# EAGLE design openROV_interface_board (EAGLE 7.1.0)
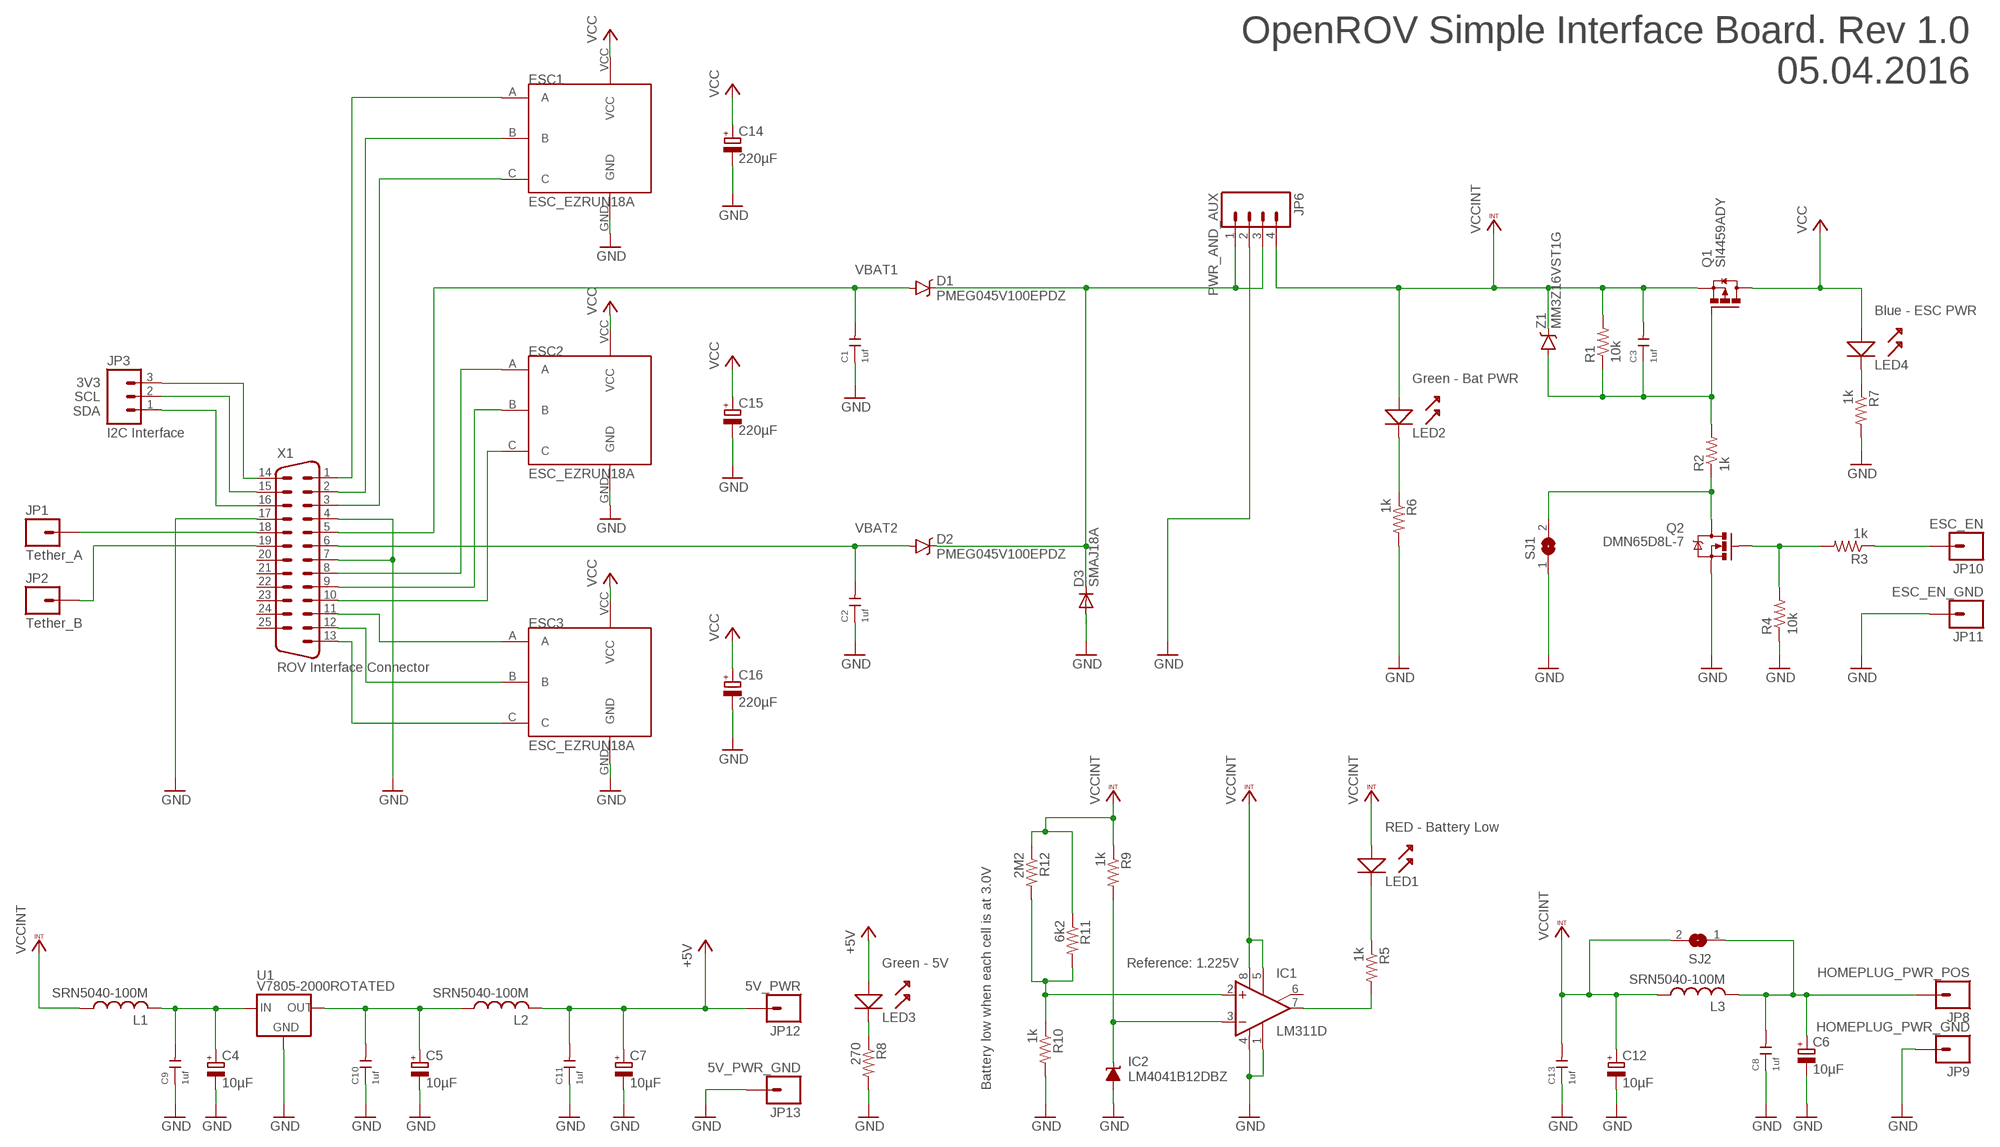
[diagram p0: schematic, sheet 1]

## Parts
C1  1uf  CERAMIC-1UF-25V-10%-X7R(0805)  [C0805]
C2  1uf  CERAMIC-1UF-25V-10%-X7R(0805)  [C0805]
C3  1uf  CERAMIC-1UF-25V-10%-X7R(0805)  [C0805]
C4  10µF  CPOL-EUE2-5  [E2-5]
C5  10µF  CPOL-EUE2-5  [E2-5]
C6  10µF  CPOL-EUE2-5  [E2-5]
C7  10µF  CPOL-EUE2-5  [E2-5]
C8  1uf  CERAMIC-1UF-25V-10%-X7R(0805)  [C0805]
C9  1uf  CERAMIC-1UF-25V-10%-X7R(0805)  [C0805]
C10  1uf  CERAMIC-1UF-25V-10%-X7R(0805)  [C0805]
C11  1uf  CERAMIC-1UF-25V-10%-X7R(0805)  [C0805]
C12  10µF  CPOL-EUE2-5  [E2-5]
C13  1uf  CERAMIC-1UF-25V-10%-X7R(0805)  [C0805]
C14  220µF  CPOL-EUE3.5-8  [E3,5-8]
C15  220µF  CPOL-EUE3.5-8  [E3,5-8]
C16  220µF  CPOL-EUE3.5-8  [E3,5-8]
D1  PMEG045V100EPDZ  [SOT1289]
D2  PMEG045V100EPDZ  [SOT1289]
D3  SMAJ18A  DIODE-DO-214AC  [DO-214AC]
ESC1  ESC_EZRUN18A  [ESC_EZRUN18A]
ESC2  ESC_EZRUN18A  [ESC_EZRUN18A]
ESC3  ESC_EZRUN18A  [ESC_EZRUN18A]
IC1  LM311D  [SO08]
IC2  LM4041B12DBZ  [DBZ_R-PDSO-G3]
JP1  Tether_A  M01PTH_LONGPAD  [1X01_LONGPAD]
JP2  Tether_B  M01PTH_LONGPAD  [1X01_LONGPAD]
JP3  I2C Interface  M03LONGPADS  [1X03_LONGPADS]
JP6  PWR_AND_AUX  M04LONGPADS  [1X04_LONGPADS]
JP8  HOMEPLUG_PWR_POS  M01PTH_LONGPAD  [1X01_LONGPAD]
JP9  HOMEPLUG_PWR_GND  M01PTH_LONGPAD  [1X01_LONGPAD]
JP10  ESC_EN  M01PTH_LONGPAD  [1X01_LONGPAD]
JP11  ESC_EN_GND  M01PTH_LONGPAD  [1X01_LONGPAD]
JP12  5V_PWR  M01PTH_LONGPAD  [1X01_LONGPAD]
JP13  5V_PWR_GND  M01PTH_LONGPAD  [1X01_LONGPAD]
L1  SRN5040-100M  [SRN5040_SERIES]
L2  SRN5040-100M  [SRN5040_SERIES]
L3  SRN5040-100M  [SRN5040_SERIES]
LED1  RED - Battery Low  LED-1206  [LED-1206]
LED2  Green - Bat PWR  LED-1206  [LED-1206]
LED3  Green - 5V  LED-1206  [LED-1206]
LED4  Blue - ESC PWR  LED-1206  [LED-1206]
Q1  SI4459ADY  [SO8]
Q2  DMN65D8L-7  [SOT-23]
R1  10k  R-US_M0805  [M0805]
R2  1k  R-US_M0805  [M0805]
R3  1k  R-US_M0805  [M0805]
R4  10k  R-US_M0805  [M0805]
R5  1k  R-US_M0805  [M0805]
R6  1k  R-US_M0805  [M0805]
R7  1k  R-US_M0805  [M0805]
R8  270  R-US_M0805  [M0805]
R9  1k  R-US_M0805  [M0805]
R10  1k  R-US_M0805  [M0805]
R11  6k2  R-US_M0805  [M0805]
R12  2M2  R-US_M0805  [M0805]
SJ1  SJW  [SJW]
SJ2  SJW  [SJW]
U1  V7805-2000ROTATED  [V78XX-2000R]
X1  ROV Interface Connector  DB25HP  [M25HP]
Z1  MM3Z16VST1G  [SOD-323]

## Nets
+5V: C7.+ C11.2 JP12.1 L2.P$2 LED3.1(A)
GND: C1.1 C2.1 C4.- C5.- C6.- C7.- C8.1 C9.1 C10.1 C11.1 C12.- C13.1 C14.- C15.- C16.- D3.A ESC1.GND ESC2.GND ESC3.GND IC1.1(GND) IC1.4(V-) IC2.2(A) JP6.2 JP9.1 JP11.1 JP13.1 Q2.2(S1) R4.1 R6.2 R7.2 R8.2 R10.2 SJ1.1 U1.P$2(GND) X1.4 X1.7 X1.17
N$1: JP1.1 X1.18
N$2: JP2.1 X1.19
N$3: JP3.3 X1.14
N$4: JP3.2 X1.15
N$5: JP3.1 X1.16
N$6: ESC3.C X1.13
N$7: ESC3.B X1.12
N$8: ESC3.A X1.11
N$9: ESC2.C X1.10
N$10: ESC2.B X1.9
N$11: ESC2.A X1.8
N$12: ESC1.A X1.1
N$13: ESC1.B X1.2
N$14: ESC1.C X1.3
N$15: D1.P$3(C) D2.P$3(C) D3.C JP6.1 JP6.3
N$16: C3.1 Q1.4(G) R1.1 R2.2 Z1.A
N$17: Q2.3(D1) R2.1 SJ1.2
N$18: Q2.1(G1) R3.2 R4.2
N$19: JP10.1 R3.1
N$20: C6.+ C8.2 JP8.1 L3.P$2 SJ2.1
N$21: C4.+ C9.2 L1.P$2 U1.P$1(IN)
N$22: C5.+ C10.2 L2.P$1 U1.P$3(OUT)
N$23: LED3.2(K) R8.1
N$24: IC1.3(-IN) IC2.1(C) R9.2
N$25: IC1.7(OUT) R5.2
N$26: LED1.2(K) R5.1
N$27: LED2.2(K) R6.1
N$28: LED4.2(K) R7.1
N$29: IC1.2(+IN) R10.1 R11.2 R12.2
VBAT1: C1.2 D1.P$1(A) D1.P$2(A) X1.5
VBAT2: C2.2 D2.P$1(A) D2.P$2(A) X1.6
VCC: C14.+ C15.+ C16.+ ESC1.VCC ESC2.VCC ESC3.VCC LED4.1(A) Q1.5(D) Q1.6(D) Q1.7(D) Q1.8(D)
VCCINT: C3.2 C12.+ C13.2 IC1.5(ON) IC1.8(V+) JP6.4 L1.P$1 L3.P$1 LED1.1(A) LED2.1(A) Q1.1(S) Q1.2(S) Q1.3(S) R1.2 R9.1 R11.1 R12.1 SJ2.2 Z1.C
Unconnected: IC1.6(ON/STR) X1.20 X1.21 X1.22 X1.23 X1.24 X1.25

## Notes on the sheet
- OpenROV Simple Interface Board. Rev 1.0
  05.04.2016
- 3V3
  SCL
  SDA
- Reference: 1.225V
- Battery low when each cell is at 3.0V

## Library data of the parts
C1-C3 C8-C11 C13 = Seeed-Capacitor-2016:CERAMIC-1UF-25V-10%-X7R(0805): 302010179; MOUSER: 603-CC805KKX7R8BB105; MPN: CC0805KKX7R8BB105
C4-C7 C12 = rcl:CPOL-EU: POLARIZED CAPACITOR, European symbol; MOUSER: 647-UPW1E100MDD
C14-C16 = rcl:CPOL-EU: POLARIZED CAPACITOR, European symbol; MOUSER: 661-EKZN350E221MH15D
D1 D2 = det_lib:PMEG045V100EPDZ; MOUSER: 771-PMEG045V100EPDZ
D3 = diode:DIODE-: DIODE; MOUSER: 511-SMAJ18A-TR
ESC1-ESC3 = uzzors2k:ESC_EZRUN18A
IC1 = linear:LM311: COMPARATOR; MOUSER: 511-LM311DT
IC2 = texas:LM4041: PRECISION MICROPOWER SHUNT VOLTAGE REFERENCE; MOUSER: 595-LM4041B12IDBZR; MPN: LM4041B12IDBZR; OC_FARNELL: 1575212; OC_NEWARK: 58K5882
JP1 JP2 JP8-JP13 = SparkFun-Connectors:M01: Header 1
JP3 = SparkFun-Connectors:M03: Header 3 Standard 3-pin 0.1" header. Use with straight break away headers (SKU : PRT-00116), right angle break away headers (PRT-00553), swiss pins (PRT-00743), machine pins (PRT-00117), and female headers (PRT-00115). Molex polarized connector foot print use with SKU : PRT-08232 with associated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
JP6 = SparkFun-Connectors:M04: Header 4 Standard 4-pin 0.1" header. Use with straight break away headers (SKU : PRT-00116), right angle break away headers (PRT-00553), swiss pins (PRT-00743), machine pins (PRT-00117), and female headers (PRT-00115). Molex polarized connector foot print use with SKU : PRT-08231 with associated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
L1-L3 = det_lib:SRN5040-100M; MOUSER: 652-SRN5040-100M
LED1 = uzzors2k:LED; MOUSER: 859-LTST-C230KRKT
LED2 LED3 = uzzors2k:LED; MOUSER: 859-LTST-C230KGKT
LED4 = uzzors2k:LED; MOUSER: 859-LTST-C230TBKT
Q1 = det_lib:SI4459ADY; MOUSER: 781-SI4459ADY-T1-GE3
Q2 = det_lib:DMN65D8L-7; MOUSER: 621-DMN65D8L-7
R1 R4 = rcl:R-US_: RESISTOR, American symbol; MOUSER: 71-CRCW0805-10K-E3
R2 R3 R5-R7 R9 R10 = rcl:R-US_: RESISTOR, American symbol; MOUSER: 588-AS08J1001ET
R8 = rcl:R-US_: RESISTOR, American symbol; MOUSER: 667-ERJ-6GEYJ271V
R11 = rcl:R-US_: RESISTOR, American symbol; MOUSER: 667-ERJ-6ENF6201V
R12 = rcl:R-US_: RESISTOR, American symbol; MOUSER: 603-RC0805FR-072M2L
SJ1 SJ2 = jumper:SJ: SMD solder JUMPER
U1 = det_lib:V7805-2000; MOUSER: 490-V7805-2000R
X1 = SparkFun-Connectors:DB25: Various DB25 connectors; MOUSER: 636-182-025-113R531
Z1 = det_lib:MM3Z16VST1G; MOUSER: 863-MM3Z16VST1G

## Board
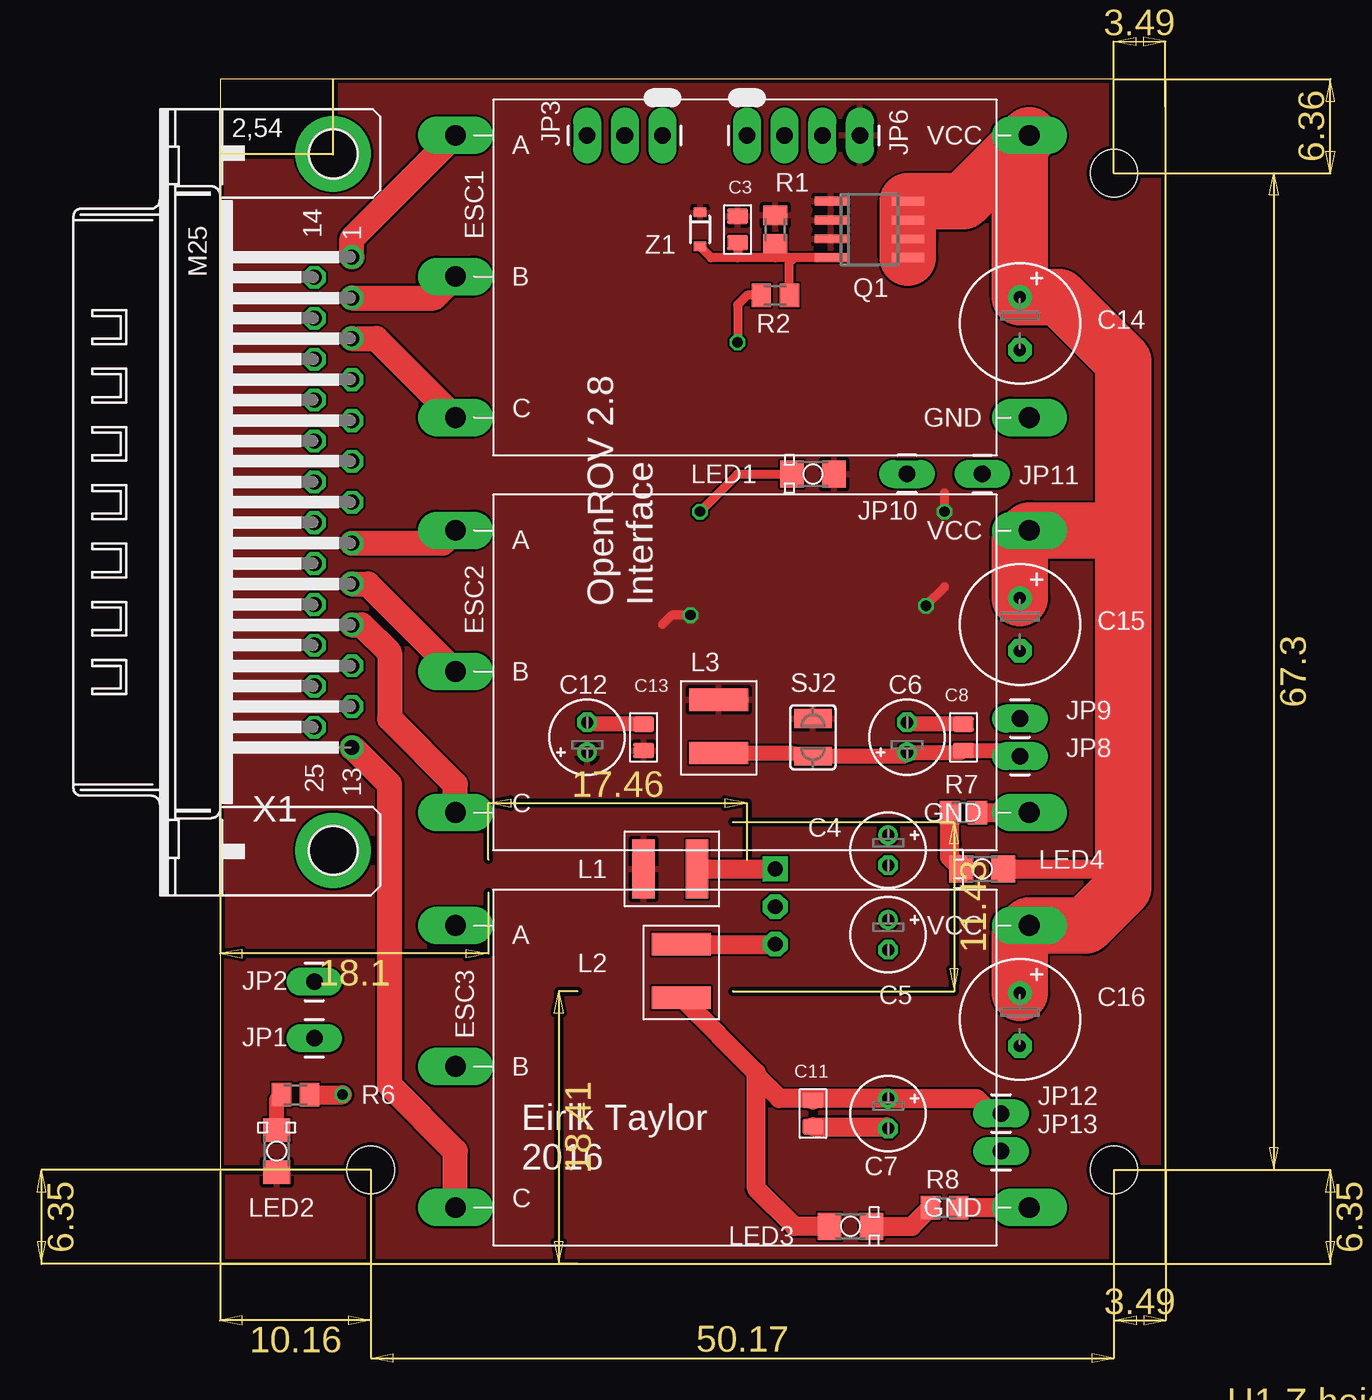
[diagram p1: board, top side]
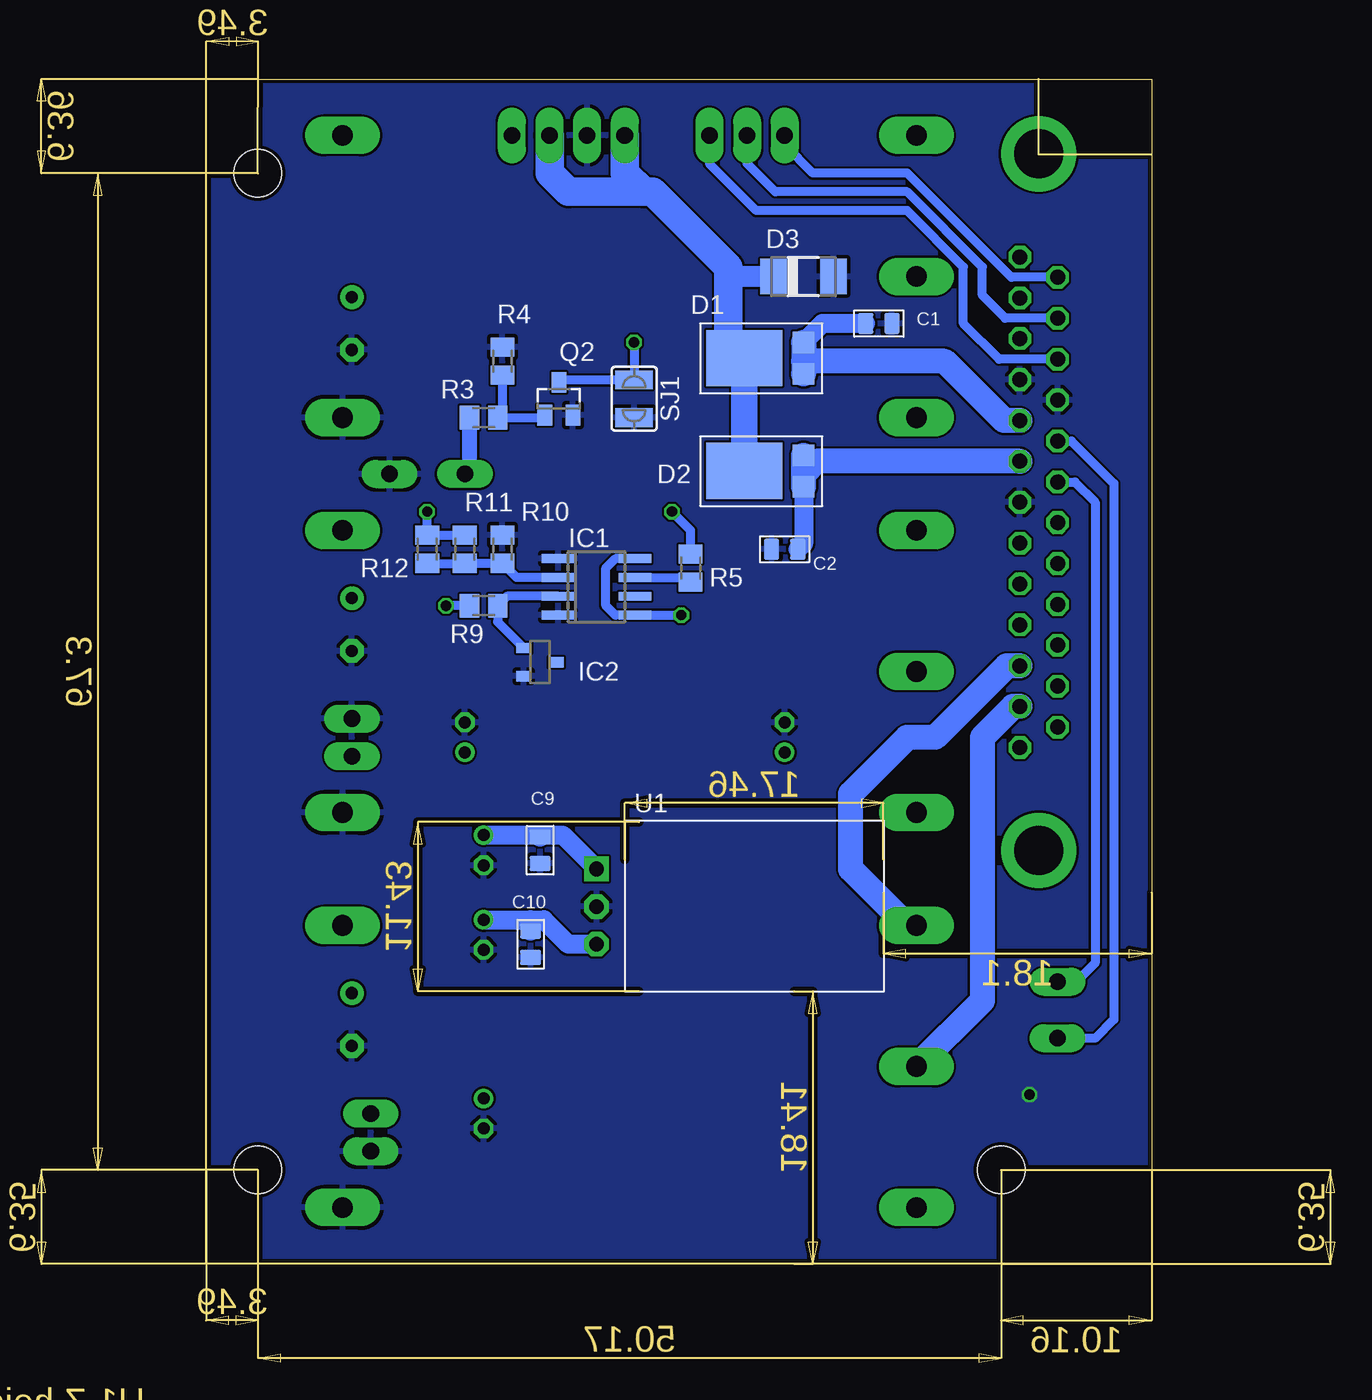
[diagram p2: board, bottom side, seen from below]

Size 87.59 x 89.49 mm. Coordinates in mm from the lower left corner, seen from the top.
Outline: 12.37,6.65 76.17,6.65 76.17,86.65 12.37,86.65 12.37,6.65
Copper layers (1*16): Top 0.035mm / dielectric 1.5mm / Bottom 0.035mm
Design rules "SeeedStudio_2layer_DRU_no_angle_20140221": minimum track width 6mil, minimum drill 12mil, track to track 6mil, track to pad 6mil, pad to pad 6mil, via to via 6mil, smd to smd 0mil, copper to edge 10mil, drill to drill 10mil, minimum pad ring 10mil, minimum via ring 6mil, stop-mask expansion 2mil, vias tented up to drill 100mil, thermal gap 10mil
Holes 3.2 mm at 22.53,13 72.69,13 72.69,80.3

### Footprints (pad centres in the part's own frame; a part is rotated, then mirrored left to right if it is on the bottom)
C0805 = smd 1.397 x 1.016: 1 0,0.889; 2 0,-0.889
E2-5 = drill 0.813 pad 1.27: + -1.016,0 | drill 0.813 pad 1.27 octagon: - 1.016,0
E3,5-8 = drill 0.813 pad 1.6: + -1.778,0 | drill 0.813 pad 1.6 octagon: - 1.778,0
SOT1289 = smd 1.44 x 1.44: P$1 -1.27,2.54; P$2 0.86,2.54 | smd 3.8 x 5.16: P$3 -0.205,-1.46
DO-214AC = smd 1.8 x 2.4: A 2.025,0; C -2.025,0
ESC_EZRUN18A = drill 1.4 pad 2.54 long: A -19.05,8.89; B -19.05,-0.635; C -19.05,-10.16; GND 19.685,-10.16; VCC 19.685,8.89
SO08 = smd 0.6 x 2.2: 1 -1.905,-2.6; 2 -0.635,-2.6; 3 0.635,-2.6; 4 1.905,-2.6; 5 1.905,2.6; 6 0.635,2.6; 7 -0.635,2.6; 8 -1.905,2.6
DBZ_R-PDSO-G3 = smd 0.7 x 1: 1 -0.95,-1.1; 2 0.95,-1.1; 3 0,1.1
1X01_LONGPAD = drill 1.118 pad 1.88 long: 1 0,0
1X03_LONGPADS = drill 1.118 pad 1.88 long: 1 0,0; 2 2.54,0; 3 5.08,0
1X04_LONGPADS = drill 1.118 pad 1.88 long: 1 0,0; 2 2.54,0; 3 5.08,0; 4 7.62,0
SRN5040_SERIES = smd 1.5 x 4: P$1 0,0; P$2 3.6,0
LED-1206 = smd 1.6 x 1.803: 1 -1.422,0; 2 1.422,0
SO8 = smd 0.6 x 2.2: 1 -1.905,-2.6; 2 -0.635,-2.6; 3 0.635,-2.6; 4 1.905,-2.6; 5 1.905,2.6; 6 0.635,2.6; 7 -0.635,2.6; 8 -1.905,2.6
SOT-23 = smd 1 x 1.4: 1 -0.95,-1.1; 2 0.95,-1.1; 3 0,1.1
M0805 = smd 1.3 x 1.6: 1 -0.95,0; 2 0.95,0
SJW = smd 1.27 x 2.54: 1 -1.27,0; 2 1.27,0
V78XX-2000R = drill 1 pad 1.676 square: P$1 -8.89,2.54 | drill 1 pad 1.676 octagon: P$2 -8.89,0; P$3 -8.89,-2.54
M25HP = drill 1.016 octagon: 1 -16.561,1.27; 2 -13.792,1.27; 3 -11.049,1.27; 4 -8.28,1.27; 5 -5.512,1.27; 6 -2.769,1.27; 7 0,1.27; 8 2.769,1.27; 9 5.512,1.27; 10 8.28,1.27; 11 11.049,1.27; 12 13.792,1.27; 13 16.561,1.27; 14 -15.189,-1.27; 15 -12.421,-1.27; 16 -9.652,-1.27; 17 -6.909,-1.27; 18 -4.14,-1.27; 19 -1.372,-1.27; 20 1.372,-1.27; 21 4.14,-1.27; 22 6.909,-1.27; 23 9.652,-1.27; 24 12.421,-1.27; 25 15.189,-1.27 | drill 3.302 pad 5.08: G1 -23.52,0; G2 23.52,0
SOD-323 = smd 0.63 x 0.83: A 1.15,0; C -1.15,0

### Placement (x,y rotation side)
C1  30.78,70.15 270 bottom
C2  37.13,54.91 90 bottom
C3  47.29,76.5 180 top
C4  57.45,34.59 270 top
C5  57.45,28.88 270 top
C6  58.72,42.21 90 top
C7  57.45,16.81 270 top
C8  62.53,42.21 0 top
C9  53.64,34.59 180 bottom
C10  54.27,28.24 180 bottom
C11  52.37,16.81 180 top
C12  37.13,42.21 90 top
C13  40.94,42.21 0 top
C14  66.34,70.15 270 top
C15  66.34,49.83 270 top
C16  66.34,23.16 270 top
D1  38.4,67.61 270 bottom
D2  38.4,59.99 270 bottom
D3  35.86,73.33 0 bottom
ESC1  47.29,73.96 0 top
ESC2  47.29,47.29 0 top
ESC3  47.29,20.62 0 top
IC1  49.83,52.37 270 bottom
IC2  53.64,47.29 270 bottom
JP1  18.72,21.89 90 top
JP2  18.72,25.7 90 top
JP3  42.21,82.85 180 top
JP6  47.93,82.85 0 top
JP8  66.34,40.94 90 top
JP9  66.34,43.48 90 top
JP10  58.72,59.99 270 top
JP11  63.8,59.99 90 top
JP12  65.07,16.81 90 top
JP13  65.07,14.27 90 top
L1  40.94,33.32 0 top
L2  43.48,28.24 270 top
L3  46.02,44.75 270 top
LED1  52.37,59.99 180 top
LED2  16.18,14.27 90 top
LED3  54.91,9.19 0 top
LED4  63.8,33.32 180 top
Q1  56.18,76.5 270 top
Q2  52.37,65.07 0 bottom
R1  49.83,76.5 90 top
R2  49.83,72.06 0 top
R3  57.45,63.8 0 bottom
R4  56.18,67.61 270 bottom
R5  43.48,53.64 270 bottom
R6  17.45,18.08 0 top
R7  62.53,37.13 0 top
R8  61.26,10.46 0 top
R9  57.45,51.1 0 bottom
R10  56.18,54.91 90 bottom
R11  58.72,54.91 270 bottom
R12  61.26,54.91 270 bottom
SJ1  47.29,65.07 90 bottom
SJ2  52.37,42.21 90 top
U1  40.94,30.78 0 bottom
X1  19.99,58.09 270 top
Z1  44.75,76.5 270 top

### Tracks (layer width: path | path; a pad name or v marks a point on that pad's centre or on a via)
+5V
  Top 1.27: 52.37,17.83 C7.+ 63.42,17.83 64.44,16.81 | L2.P$2 48.56,19.56 48.56,19.35 | C11.2 52.37,17.83 | JP12.1 64.44,16.81 | 64.44,16.81 63.8,16.81 | LED3.1 51.1,9.19 48.56,11.73 48.56,19.35 | 52.37,17.83 50.08,17.83 48.56,19.35
GND  (via drill 0.7)
  Top 1.016: C13.1 37.26,43.1 C12.- | C8.1 58.85,43.1 C6.-
  Top 1.27: C11.1 57.32,15.92 C7.- | R8.2 ESC3.GND | R6.2 v20.62,18.08 | R7.2 ESC2.GND
  pour Bottom: 12.37,86.66 100,86.66 100,6.65 12.37,6.65
N$1
  Bottom 0.61: X1.18 17.78,62.23 14.91,59.35 14.91,23.16 16.18,21.89 JP1.1
N$2
  Bottom 0.61: X1.19 17.55,59.46 16.18,58.09 16.18,26.97 17.45,25.7 JP2.1
N$3
  Bottom 0.61: X1.14 21.84,73.27 28.88,80.31 35.23,80.31 37.13,82.22 JP3.3
N$4
  Bottom 0.61: X1.15 22.25,70.51 23.8,72.06 23.8,73.96 28.88,79.04 37.77,79.04 39.67,80.95 JP3.2
N$5
  Bottom 0.61: X1.16 22.65,67.74 25.07,70.15 25.07,73.96 28.88,77.77 39.04,77.77 42.21,80.95 JP3.1
N$6
  Top 1.676: X1.13 21.31,41.52 23.8,39.03 23.8,18.71 28.24,14.27 ESC3.C
N$7
  Bottom 1.676: X1.12 21.71,44.29 23.8,42.21 23.8,24.43 ESC3.B
N$8
  Bottom 1.676: ESC3.A 28.88,29.51 32.69,33.32 32.69,38.4 28.88,42.21 26.97,42.21 22.14,47.04 X1.11
N$9
  Top 1.676: X1.10 21.92,49.8 23.8,47.92 23.8,43.48 28.24,39.03 ESC2.C
N$10
  Top 1.676: X1.9 22.32,52.57 ESC2.B
N$11
  Top 1.676: X1.8 27.38,55.32 ESC2.A
N$12
  Top 1.676: X1.1 21.26,75.87 ESC1.A
N$13
  Top 1.676: X1.2 26.79,71.88 ESC1.B
N$14
  Top 1.676: X1.3 22.91,69.13 ESC1.C
N$15
  Bottom 1.422: D3.C 40.31,73.33 40.94,73.96
  Bottom 1.778: D1.P$3 D2.P$3
  Bottom 1.93: D1.P$3 40.94,68.89 40.94,73.96 46.02,79.04 46.66,79.04 | 46.66,79.04 51.73,79.04 53.01,80.31 JP6.3 | JP6.1 47.93,80.31 46.66,79.04
N$16
  Top 0.61: Q1.4 51.1,74.59 | 51.1,74.59 49.83,74.59 | 49.83,74.59 47.29,74.59 | 47.29,74.59 45.51,74.59 Z1.A | R2.2 50.78,74.28 51.1,74.59 | R1.1 49.83,74.59 | C3.1 47.29,74.59
N$17  (via drill 0.7)
  Top 0.61: R2.1 47.93,72.06 47.29,71.42 v47.29,68.88
  Bottom 0.61: Q2.3 52.2,66.34 SJ1.2 v47.29,68.88
N$18
  Bottom 0.61: Q2.1 53.49,63.8 R3.2 56.18,64.12 R4.2
N$19
  Bottom 1.016: JP10.1 58.4,59.99 R3.1
N$20
  Top 1.016: 45.85,41.32 L3.P$2 50.89,41.15 SJ2.1 58.47,40.94 C6.+ 62.4,41.19 C8.2 65.96,41.32 JP8.1
N$21
  Top 1.27: L1.P$2 U1.P$1
  Bottom 1.27: C4.+ 53.64,35.61 | 53.64,35.61 52.12,35.61 U1.P$1 | C9.2 53.64,35.61
N$22
  Top 1.27: L2.P$1 U1.P$3
  Bottom 1.27: C5.+ 54.27,29.89 | 54.27,29.89 53.39,29.89 51.73,28.24 U1.P$3 | C10.2 54.27,29.89
N$23
  Top 1.27: LED3.2 59.04,9.19 R8.1
N$24
  Bottom 0.61: IC1.3 55.87,51.73 R9.2 56.5,50 IC2.1
N$25
  Bottom 0.61: IC1.7 43.8,53 R5.2
N$26  (via drill 0.7)
  Top 0.61: v44.75,57.45 47.29,59.99 LED1.2
  Bottom 0.61: R5.1 43.48,56.18 v44.75,57.45
N$27
  Top 1.016: LED2.2 16.18,17.76 R6.1
N$28
  Top 1.27: R7.1 61.58,34.12 LED4.2
N$29
  Bottom 0.61: IC1.2 55.23,53 R10.1 R11.2 R12.2
VBAT1
  Bottom 1.27: C1.2 34.59,70.15 D1.P$1
  Bottom 1.676: D1.P$1 35.86,67.61 | 35.86,67.61 D1.P$2 | X1.5 22.32,63.6 26.34,67.61 35.86,67.61
VBAT2
  Bottom 1.27: D2.P$2 35.86,55.29 C2.2
  Bottom 1.676: D2.P$2 35.86,59.99 | 35.86,59.99 D2.P$1 | X1.6 35,60.85 35.86,59.99
VCC
  Top 1.27: LED4.1 73.33,33.32
  Top 3.81: Q1.5 Q1.6 Q1.7 Q1.8 62.53,78.41 ESC1.VCC 66.34,82.22 C14.+ 69.01,71.93 73.33,67.61 73.33,56.18 | 73.33,56.18 73.33,33.32 73.33,32.05 70.78,29.51 ESC3.VCC 66.34,28.88 C16.+ | 73.33,56.18 ESC2.VCC 66.34,55.55 C15.+
VCCINT  (via drill 0.7)
  Top 0.61: v59.99,51.1 61.26,52.37 | v61.26,57.45 61.26,58.72 | v44.12,50.46 42.84,50.46 42.21,49.83
  Bottom 0.61: IC1.8 48.56,54.27 49.2,53.64 49.2,51.1 48.56,50.46 IC1.5 v44.12,50.46 | R11.1 R12.1 v61.26,57.45 | R9.1 v59.99,51.1
  pour Top: 12.37,86.66 88.56,86.66 88.56,6.65 12.37,6.65

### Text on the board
Dimension: U1 Z height: 9.0mm
tNames: OpenROV 2.8 / Interface | Eirik Taylor / 2016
